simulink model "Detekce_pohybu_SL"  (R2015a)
settings: Solver=ode45  StartTime=0.0  StopTime=10.0  RelTol=1e-3
undefined symbols (not defined in the file or in its folder): adaptor, C, genericvideo, HD, HP, imaq, IsPositionTracked, IsSkeletonTracked, JointDepthIndices, JointImageIndices, JointTrackingState, JointWorldCoordinates, MATLAB, osgenericvideointerface, PositionDepthIndices, PositionImageIndices, PositionWorldCoordinates, R2015a, Rec, SDTV, SegmentationData, SkeletonTrackingID, SupportPackages, supportpackages, toolbox, videoinput, Webcam, win64, winvideo
libraries: visionconversions x1, imaqlib x1, visionsinks x1

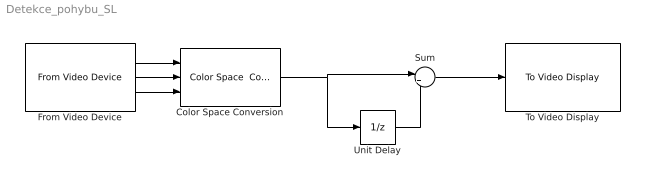
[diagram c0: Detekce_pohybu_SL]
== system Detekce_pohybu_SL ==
  Color Space Conversion : visionconversions/Color Space  Conversion  conversion=Obsolete  conversionActive=R'G'B' to intensity  wp_str=D65  rec=Rec. 601 (SDTV)  sys=1125/60/2:1  imagePorts=Separate color signals
  From Video Device : imaqlib/From Video Device  DeviceMenu=winvideo 1 (HP HD Webcam)  Device=winvideo 1 (HP HD Webcam)  ObjConstructor=videoinput('winvideo', 1)  VideoFormatMenu=RGB24_640x480  VideoFormat=RGB24_640x480  VideoSource=input1  ROIPosition=[0 0 480 640]  EnableHWTrigger=off  TriggerConfiguration=winvideo 1 (HP HD Webcam)  SampleTime=1/30  OutputPortsMode=Separate color signals  DataType=uint8  CanDoHWTrigger=no  ReturnedColorSpace=rgb  BlockHandle=1975.0006  ROIWidth=640  ROIHeight=480  ROIColumn=0  ROIRow=0  EngXMLPath=C:\Program Files\MATLAB\R2015a\toolbox\imaq\imaq\private  DevXMLPath=C:\MATLAB\SupportPackages\R2015a\osgenericvideointerface\toolbox\imaq\supportpackages\genericvideo\adaptor\win64  EngLibPath=C:\Program Files\MATLAB\R2015a\toolbox\imaq\imaqblks\imaqmex\win64  ColorSpace=rgb  BayerSensorAlignment=grbg  AllMetadata=IsPositionTracked;IsSkeletonTracked;JointDepthIndices;JointImageIndices;JointTrackingState;JointWorldCoordinates;PositionDepthIndices;PositionImageIndices;PositionWorldCoordinates;SegmentationData;SkeletonTrackingID
  Sum : Sum  Inputs=|+-
  To Video Display : visionsinks/To Video Display  windowSizeMode=Normal  openAtMdlStart=on  fullScreen=off  videoWindowX=610  videoWindowY=280  saveWindowSize=off  videoWindowWidth=640  videoWindowHeight=480  inputColorFormat=RGB  inputType=Obsolete  imagePorts=One multidimensional signal  OutputDevice=On-screen video monitor  dataOrg=Column-major  isWindowOpen=off
  Unit Delay : UnitDelay  SampleTime=-1
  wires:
  From Video Device/3 -> Color Space Conversion/3
  From Video Device/2 -> Color Space Conversion/2
  From Video Device/1 -> Color Space Conversion/1
  Color Space Conversion/1 -> Sum/1, Unit Delay/1
  Sum/1 -> To Video Display/1
  Unit Delay/1 -> Sum/2
